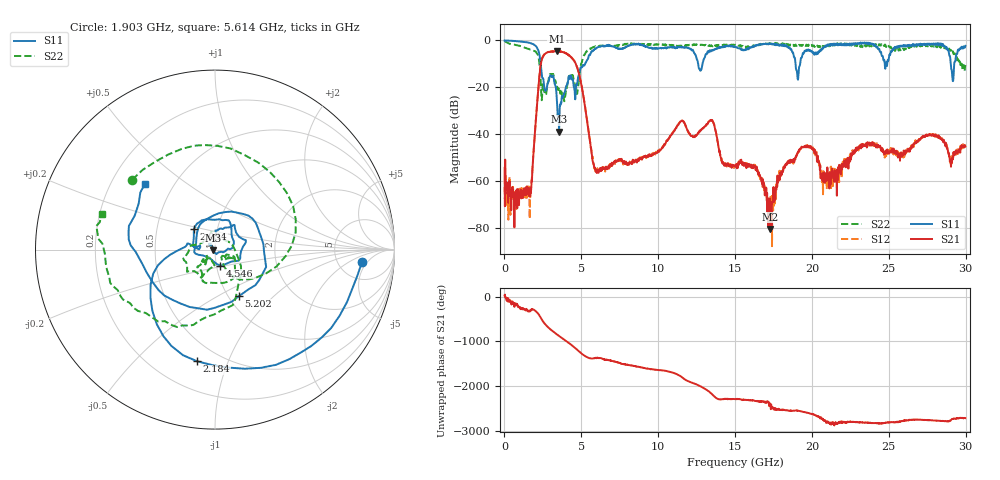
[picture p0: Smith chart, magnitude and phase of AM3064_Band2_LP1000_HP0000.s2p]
# Hz S DB R 50.0
!freq dBS11 angS11 dBS21 angS21 dBS12 angS12 dBS22 angS22
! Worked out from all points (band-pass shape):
!   1600 points, 10 MHz to 29.98 GHz, reference 50 ohm
!   highest |S21| = -4.47 dB at 3.403 GHz (marker M1); lowest = -80.4 dB at 17.25 GHz (marker M2)
!   |S21| within 3 dB of the highest: 2.46 GHz to 4.382 GHz (1.922 GHz wide, 56.2 % of centre)
!   lowest |S11| = -38.9 dB at 3.553 GHz (marker M3), VSWR 1.02, Z = 48.9 - j0.333 ohm
!   |S11| at or under -10 dB: 2.359 GHz to 5.246 GHz (2.888 GHz wide, 75.9 % of centre); 12.6 GHz to 12.88 GHz (280.9 MHz wide, 2.2 % of centre); 18.93 GHz to 19.23 GHz (301.8 MHz wide, 1.58 % of centre)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
!   |S22| runs from -26.0 to -0.2 dB; largest |S21 - S12| = 0.012
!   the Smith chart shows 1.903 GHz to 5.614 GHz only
!   S11 on the Smith chart (normalised r, x): 1.903 GHz: 8.56, -3.73; 2.184 GHz: 0.38, -0.78; 2.934 GHz: 0.77, +0.18; 4.546 GHz: 1.05, -0.19; 5.202 GHz: 1.12, -0.63; 5.614 GHz: 0.35, +0.35
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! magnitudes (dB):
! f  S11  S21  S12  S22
! 10 MHz  0.0  -54.4  -62.7  -0.2
! 1.566 GHz  -0.9  -62.9  -63.3  -3.6
! 1.903 GHz  -1.7  -46.7  -46.5  -4.4
! 2.184 GHz  -4.0  -22.0  -22.0  -6.4
! 2.54 GHz  -17.1  -6.5  -6.4  -19.4
! 2.934 GHz  -15.7  -4.9  -4.9  -14.8
! 3.403 GHz  -24.7  -4.5  -4.6  -19.9
! 3.553 GHz  -38.9  -4.8  -4.7  -20.2
! 4.546 GHz  -20.5  -8.8  -8.8  -17.3
! 5.015 GHz  -11.5  -19.3  -19.3  -9.6
! 5.202 GHz  -10.7  -26.6  -26.4  -6.2
! 5.614 GHz  -5.4  -45.9  -45.3  -3.6
! 6.064 GHz  -2.9  -56.0  -55.5  -2.4
! 10 GHz  -3.4  -47.0  -47.0  -1.8
! 13.43 GHz  -4.6  -34.0  -33.9  -2.5
! 15 GHz  -2.5  -53.8  -53.6  -1.8
! 16.35 GHz  -2.2  -55.1  -54.1  -2.4
! 17.25 GHz  -1.4  -80.4  -74.8  -1.2
! 19.99 GHz  -4.5  -45.7  -46.3  -1.9
! 20.83 GHz  -2.9  -60.8  -60.1  -2.3
! 25 GHz  -7.9  -47.9  -46.5  -2.3
! 29.98 GHz  -2.3  -45.2  -45.2  -10.5
